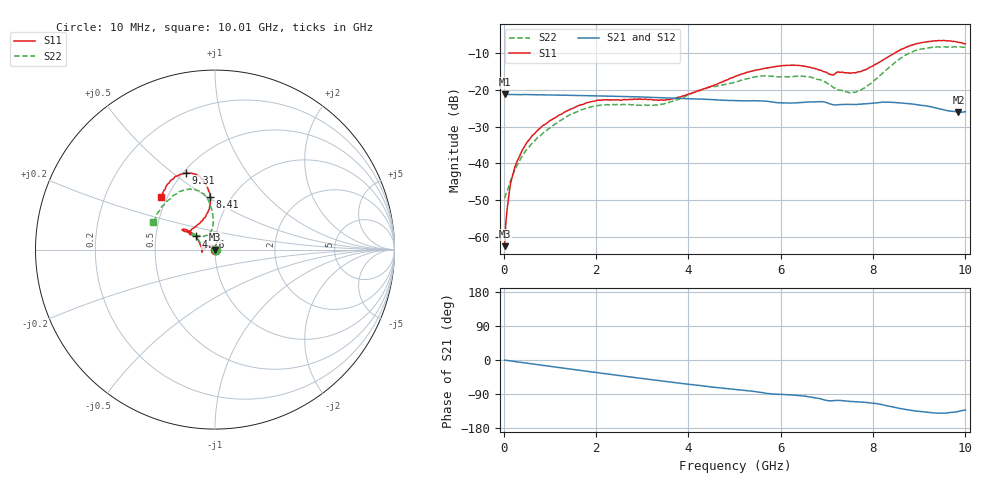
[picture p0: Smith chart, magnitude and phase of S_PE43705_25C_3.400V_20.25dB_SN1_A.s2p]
! Device ID: PE43705
! Serial: 1
! Insertion: A
! Impedance: 50 ohm
! Temp: 25C
! VDD: 3.400V
! Attenuation Step: 20.25dB
#  Hz  S  RI  R  50
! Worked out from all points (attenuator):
!   401 points, 10 MHz to 10.01 GHz, reference 50 ohm
!   highest |S21| = -21.29 dB at 10 MHz (marker M1); lowest = -26.1 dB at 9.86 GHz (marker M2)
!   lowest |S11| = -62.4 dB at 10 MHz (marker M3), VSWR 1.00, Z = 49.9 + j0.0396 ohm
!   |S11| at or under -10 dB: start of sweep to 8.484 GHz
!   |S22| runs from -49.4 to -8.4 dB; largest |S21 - S12| = 0.00098
!   S11 on the Smith chart (normalised r, x): 10 MHz: 1.00, +0.00; 4.76 GHz: 0.80, +0.12; 8.41 GHz: 0.80, +0.52; 9.31 GHz: 0.52, +0.56; 10.01 GHz: 0.47, +0.33
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1e7  -0.000646 0.000396  0.0862 -0.000402  0.0862 -0.000361  0.00336 0.000365
8.5e7  -0.000408 0.00302  0.0859 -0.00233  0.0859 -0.00227  0.00373 0.00265
1.6e8  -0.000885 0.00599  0.0858 -0.00426  0.0858 -0.0042  0.00331 0.00535
2.6e8  -0.0022 0.00969  0.0854 -0.0068  0.0854 -0.00673  0.00202 0.0087
4.35e8  -0.00595 0.0155  0.0851 -0.0112  0.0847 -0.011  -0.00139 0.0137
8.35e8  -0.023 0.0229  0.0824 -0.0207  0.0824 -0.0206  -0.0165 0.0194
1.685e9  -0.0618 0.00965  0.0734 -0.039  0.0733 -0.0389  -0.0527 0.00879
2.16e9  -0.0726 -0.00502  0.0666 -0.0477  0.0666 -0.0476  -0.0616 -0.00132
3.36e9  -0.0716 -0.00419  0.0452 -0.0635  0.0453 -0.0633  -0.0617 0.00859
4.76e9  -0.1063 0.0736  0.0193 -0.0693  0.0192 -0.0692  -0.0968 0.0653
5.01e9  -0.1218 0.0886  0.0152 -0.0694  0.0152 -0.0694  -0.1042 0.0728
5.985e9  -0.1768 0.1133  -0.000736 -0.0661  -0.000571 -0.066  -0.1197 0.0885
6.685e9  -0.1686 0.1011  -0.0101 -0.0673  -0.0102 -0.0675  -0.1203 0.0799
7.11e9  -0.1336 0.0863  -0.0192 -0.0602  -0.019 -0.06  -0.082 0.0757
7.585e9  -0.0936 0.1419  -0.0215 -0.0591  -0.0212 -0.0591  -0.0378 0.084
7.885e9  -0.0519 0.1843  -0.0247 -0.0595  -0.0244 -0.0599  -0.0179 0.1117
8.36e9  -0.025 0.2837  -0.0357 -0.0573  -0.0357 -0.0574  -0.0139 0.2013
8.41e9  -0.0278 0.2955  -0.0369 -0.0563  -0.0368 -0.0563  -0.0167 0.212
8.86e9  -0.077 0.396  -0.0437 -0.0464  -0.0436 -0.0467  -0.0758 0.3166
9.31e9  -0.1626 0.4266  -0.044 -0.0373  -0.044 -0.0374  -0.1735 0.3325
9.86e9  -0.2766 0.337  -0.0354 -0.0345  -0.0356 -0.0345  -0.3116 0.2135
1.001e10  -0.2994 0.2921  -0.0336 -0.0373  -0.0339 -0.0374  -0.3445 0.1525
